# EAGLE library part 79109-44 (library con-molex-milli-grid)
RECEPTACAL
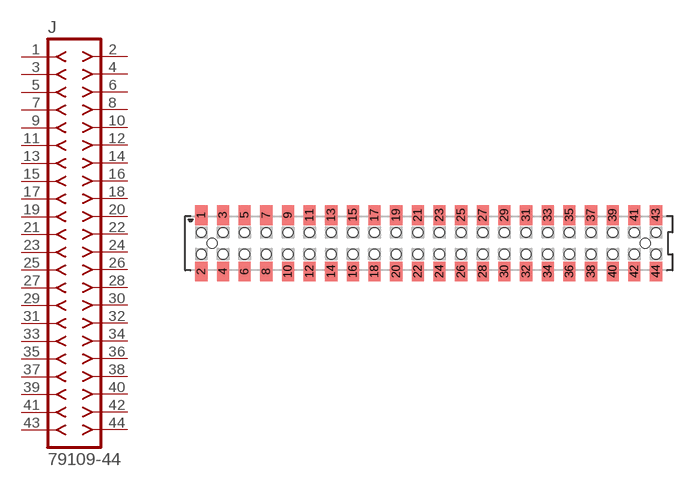
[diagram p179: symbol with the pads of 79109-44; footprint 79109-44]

Designator prefix J

## 79109-44  [79109-44]
1  1  pas
2  2  pas
3  3  pas
4  4  pas
5  5  pas
6  6  pas
7  7  pas
8  8  pas
9  9  pas
10  10  pas
11  11  pas
12  12  pas
13  13  pas
14  14  pas
15  15  pas
16  16  pas
17  17  pas
18  18  pas
19  19  pas
20  20  pas
21  21  pas
22  22  pas
23  23  pas
24  24  pas
25  25  pas
26  26  pas
27  27  pas
28  28  pas
29  29  pas
30  30  pas
31  31  pas
32  32  pas
33  33  pas
34  34  pas
35  35  pas
36  36  pas
37  37  pas
38  38  pas
39  39  pas
40  40  pas
41  41  pas
42  42  pas
43  43  pas
44  44  pas

## Footprint 79109-44 (pad centres in mm)
RECEPTACAL SMD Dual Row, Vertical, Pass-Thru
smd 1.12 x 1.83: 1 -21,2.6; 2 -21,-2.6; 3 -19,2.6; 4 -19,-2.6; 5 -17,2.6; 6 -17,-2.6; 7 -15,2.6; 8 -15,-2.6; 9 -13,2.6; 10 -13,-2.6; 11 -11,2.6; 12 -11,-2.6; 13 -9,2.6; 14 -9,-2.6; 15 -7,2.6; 16 -7,-2.6; 17 -5,2.6; 18 -5,-2.6; 19 -3,2.6; 20 -3,-2.6; 21 -1,2.6; 22 -1,-2.6; 23 1,2.6; 24 1,-2.6; 25 3,2.6; 26 3,-2.6; 27 5,2.6; 28 5,-2.6; 29 7,2.6; 30 7,-2.6; 31 9,2.6; 32 9,-2.6; 33 11,2.6; 34 11,-2.6; 35 13,2.6; 36 13,-2.6; 37 15,2.6; 38 15,-2.6; 39 17,2.6; 40 17,-2.6; 41 19,2.6; 42 19,-2.6; 43 21,2.6; 44 21,-2.6
hole 0.914 at -20,0
hole 0.914 at -21,1
hole 0.914 at -21,-1
hole 0.914 at -19,-1
hole 0.914 at -19,1
hole 0.914 at -17,-1
hole 0.914 at -17,1
hole 0.914 at 20,0
hole 0.914 at -15,1
hole 0.914 at -15,-1
hole 0.914 at -13,1
hole 0.914 at -13,-1
hole 0.914 at -11,1
hole 0.914 at -11,-1
hole 0.914 at -9,1
hole 0.914 at -9,-1
hole 0.914 at -7,-1
hole 0.914 at -7,1
hole 0.914 at -5,1
hole 0.914 at -5,-1
hole 0.914 at -3,1
hole 0.914 at -3,-1
hole 0.914 at -1,1
hole 0.914 at -1,-1
hole 0.914 at 1,-1
hole 0.914 at 1,1
hole 0.914 at 3,1
hole 0.914 at 5,1
hole 0.914 at 7,1
hole 0.914 at 3,-1
hole 0.914 at 5,-1
hole 0.914 at 7,-1
hole 0.914 at 9,-1
hole 0.914 at 11,-1
hole 0.914 at 13,-1
hole 0.914 at 15,-1
hole 0.914 at 17,-1
hole 0.914 at 9,1
hole 0.914 at 11,1
hole 0.914 at 13,1
hole 0.914 at 15,1
hole 0.914 at 17,1
hole 0.914 at 19,-1
hole 0.914 at 21,-1
hole 0.914 at 19,1
hole 0.914 at 21,1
